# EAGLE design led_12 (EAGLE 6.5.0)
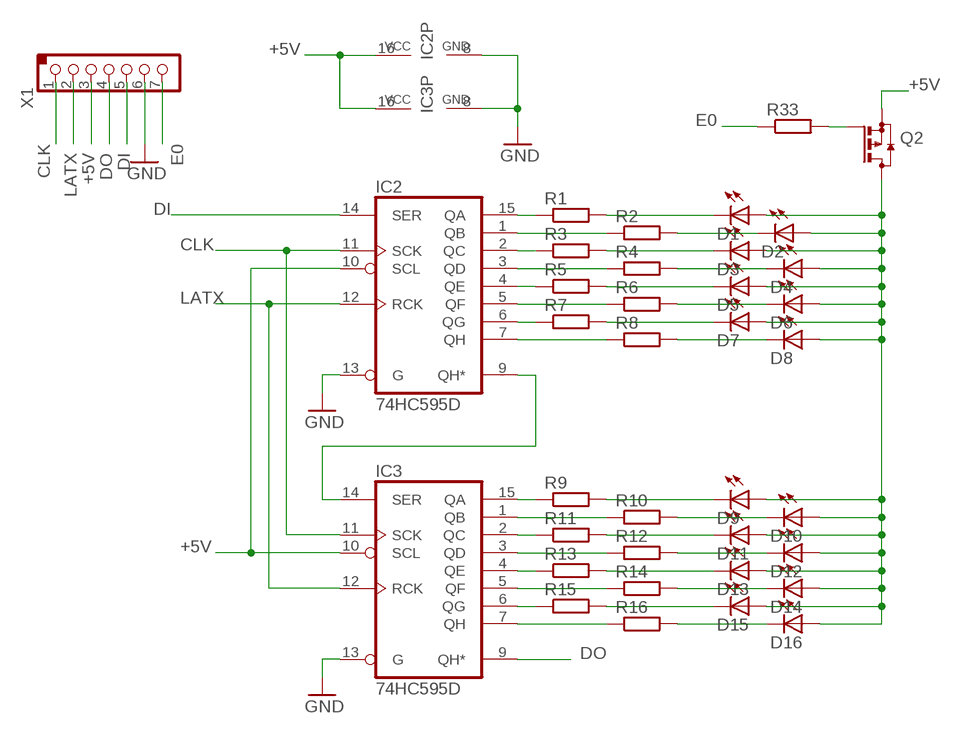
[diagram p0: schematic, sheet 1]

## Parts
D1  LED-SH  [LED5MM_SH]
D2  LED-SH  [LED5MM_SH]
D3  LED-SH  [LED5MM_SH]
D4  LED-SH  [LED5MM_SH]
D5  LED-SH  [LED5MM_SH]
D6  LED-SH  [LED5MM_SH]
D7  LED-SH  [LED5MM_SH]
D8  LED-SH  [LED5MM_SH]
D9  LED-SH  [LED5MM_SH]
D10  LED-SH  [LED5MM_SH]
D11  LED-SH  [LED5MM_SH]
D12  LED-SH  [LED5MM_SH]
D13  LED-SH  [LED5MM_SH]
D14  LED-SH  [LED5MM_SH]
D15  LED-SH  [LED5MM_SH]
D16  LED-SH  [LED5MM_SH]
IC2  74HC595D  [SO16]
IC3  74HC595D  [SO16]
Q2  BSS84  [SOT23]
R1  R_EU-0805  [SMD_0805]
R2  R_EU-0805  [SMD_0805]
R3  R_EU-0805  [SMD_0805]
R4  R_EU-0805  [SMD_0805]
R5  R_EU-0805  [SMD_0805]
R6  R_EU-0805  [SMD_0805]
R7  R_EU-0805  [SMD_0805]
R8  R_EU-0805  [SMD_0805]
R9  R_EU-0805  [SMD_0805]
R10  R_EU-0805  [SMD_0805]
R11  R_EU-0805  [SMD_0805]
R12  R_EU-0805  [SMD_0805]
R13  R_EU-0805  [SMD_0805]
R14  R_EU-0805  [SMD_0805]
R15  R_EU-0805  [SMD_0805]
R16  R_EU-0805  [SMD_0805]
R33  R_EU-1206  [SMD_1206]
X1  PINH_1X7/2  [1X7/2,0]

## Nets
+5V: IC2.10(SCL) IC2.16(VCC) IC3.10(SCL) IC3.16(VCC) Q2.2(S) X1.3
CLK: IC2.11(SCK) IC3.11(SCK) X1.1
DI: IC2.14(SER) X1.5
DO: IC3.9(QH*) X1.4
E0: R33.1 X1.7
GND: IC2.8(GND) IC2.13(G) IC3.8(GND) IC3.13(G) X1.6
LATX: IC2.12(RCK) IC3.12(RCK) X1.2
N$26: IC2.9(QH*) IC3.14(SER)
N$27: IC2.15(QA) R1.1
N$28: IC2.1(QB) R2.1
N$29: IC2.2(QC) R3.1
N$30: IC2.3(QD) R4.1
N$31: IC2.4(QE) R5.1
N$32: IC2.5(QF) R6.1
N$33: IC2.6(QG) R7.1
N$34: IC2.7(QH) R8.1
N$35: D1.C R1.2
N$36: D2.C R2.2
N$37: D3.C R3.2
N$38: D4.C R4.2
N$39: D5.C R5.2
N$40: D6.C R6.2
N$41: D7.C R7.2
N$42: D8.C R8.2
N$43: IC3.15(QA) R9.1
N$44: D9.C R9.2
N$45: IC3.1(QB) R10.1
N$46: D10.C R10.2
N$47: IC3.2(QC) R11.1
N$48: D11.C R11.2
N$49: IC3.3(QD) R12.1
N$50: D12.C R12.2
N$51: IC3.4(QE) R13.1
N$52: D13.C R13.2
N$53: IC3.5(QF) R14.1
N$54: D14.C R14.2
N$55: IC3.6(QG) R15.1
N$56: D15.C R15.2
N$57: IC3.7(QH) R16.1
N$58: D16.C R16.2
N$72: D1.A D2.A D3.A D4.A D5.A D6.A D7.A D8.A D9.A D10.A D11.A D12.A D13.A D14.A D15.A D16.A Q2.3(D)
N$73: Q2.1(G) R33.2

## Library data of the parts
D1-D16 = _dpa222:LED
IC2 IC3 = 74xx-eu:74*595: 8-bit SHIFT REGISTER, output latch
Q2 = transistor-small-signal:BSS84: P-CHANNEL MOS FET
R1-R16 R33 = _dpa222:R_EU
X1 = _dpa222:PINH_1X7/2

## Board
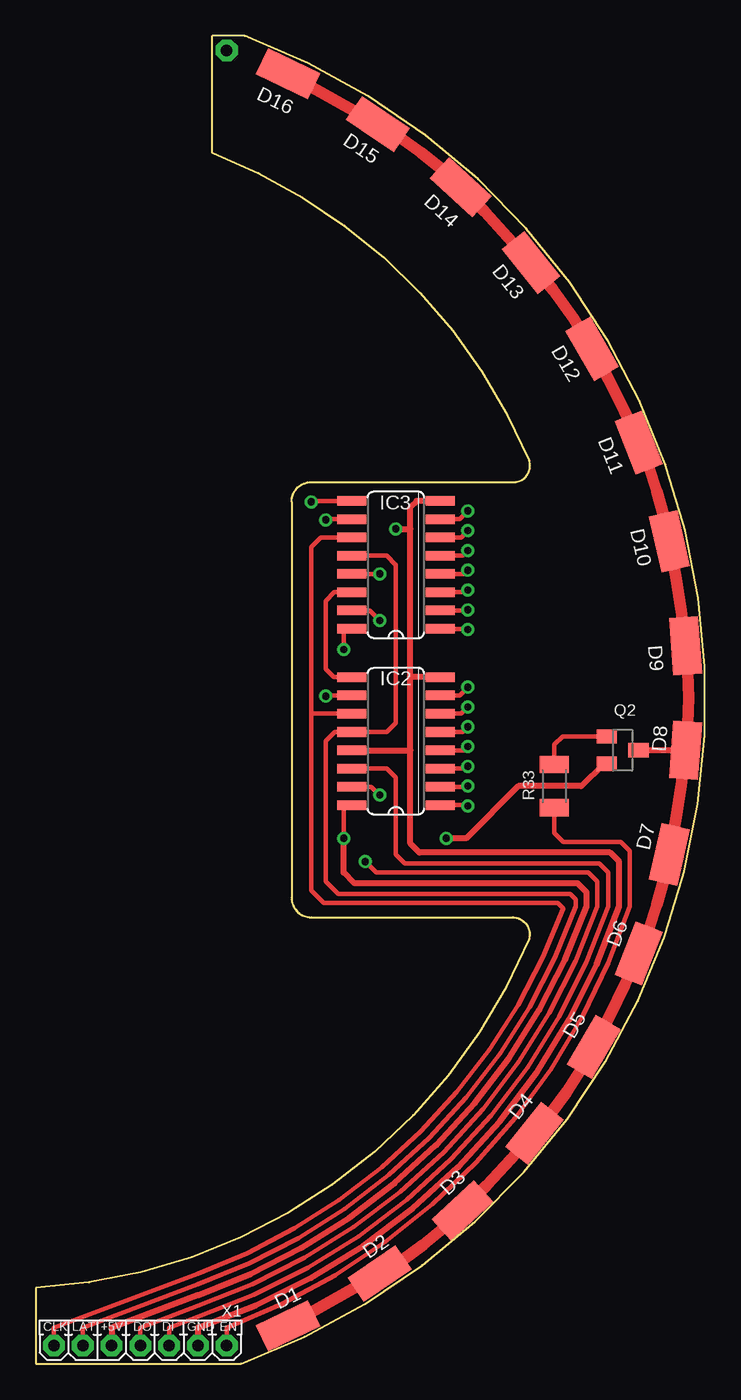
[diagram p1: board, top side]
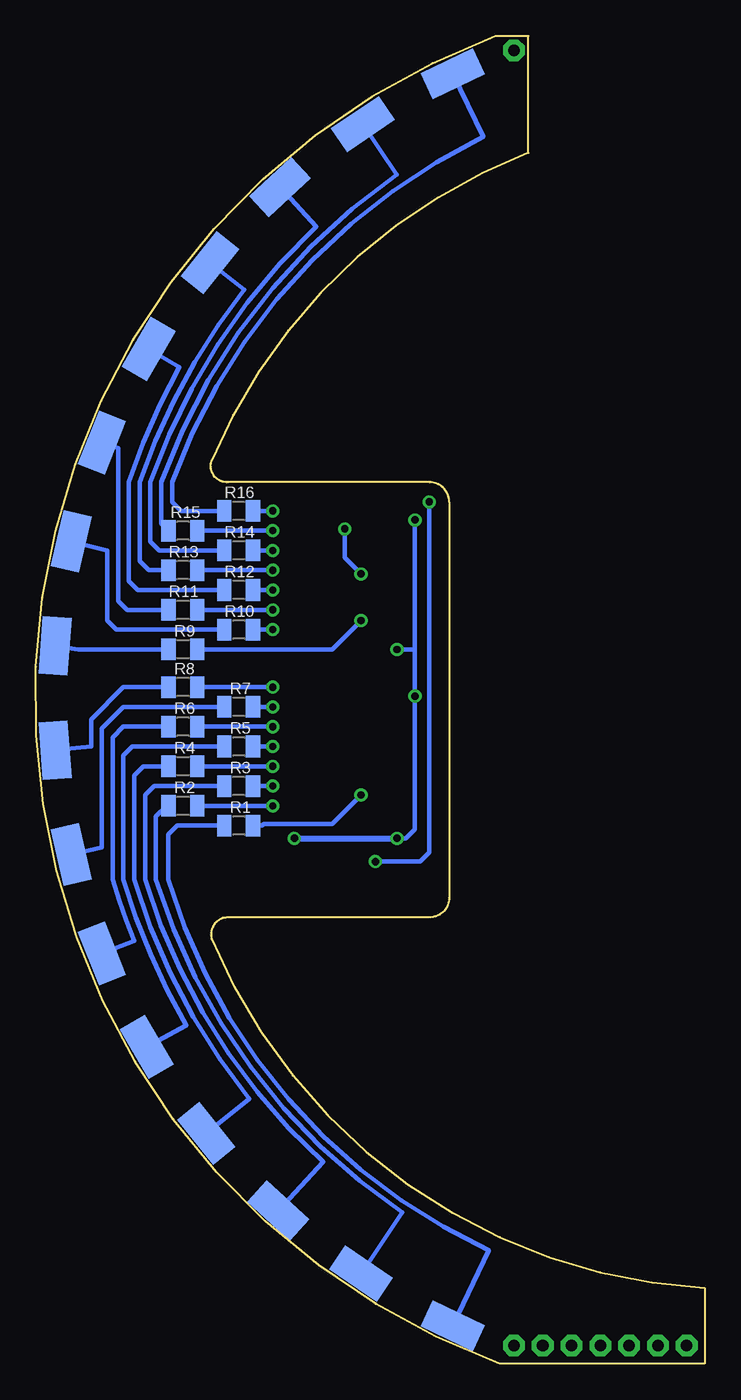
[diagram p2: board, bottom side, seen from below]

Size 46.45 x 92.25 mm. Coordinates in mm from the lower left corner, seen from the top.
Outline: 14.25,0 arc139 14.5,92.25 12.25,92.25 12.25,84.12 arc-46 34.25,62.75 arc-113 33.12,61.25 19.12,61.25 arc90 17.75,59.88 17.75,32.38 arc90 19.12,31 33.12,31 arc-106 34.25,29.5 arc-64 0,5.25 0,0 14.25,0
Copper layers (1*16): Top 0.035mm / dielectric 1.5mm / Bottom 0.035mm
Design rules "default *": minimum track width 10mil, minimum drill 24mil, track to track 8mil, track to pad 8mil, pad to pad 8mil, via to via 8mil, smd to smd 8mil, copper to edge 40mil, drill to drill 8mil, minimum pad ring 10mil, minimum via ring 8mil, stop-mask expansion 4mil, vias tented up to drill 0mil, thermal gap 10mil

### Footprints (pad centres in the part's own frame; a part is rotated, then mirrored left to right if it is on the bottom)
LED5MM_SH = smd 2 x 4: A 0,0 | smd 2 x 4 bottom: C 0,0
SO16 = smd 0.66 x 2.032: 1 -4.445,-3.073; 2 -3.175,-3.073; 3 -1.905,-3.073; 4 -0.635,-3.073; 5 0.635,-3.073; 6 1.905,-3.073; 7 3.175,-3.073; 8 4.445,-3.073; 9 4.445,3.073; 10 3.175,3.073; 11 1.905,3.073; 12 0.635,3.073; 13 -0.635,3.073; 14 -1.905,3.073; 15 -3.175,3.073; 16 -4.445,3.073
SOT23 = smd 1 x 1.4: 1 -0.95,-1.1; 2 0.95,-1.1; 3 0,1.1
SMD_0805 = smd 1 x 1.5: 1 -1,0; 2 1,0
SMD_1206 = smd 1.2 x 2: 1 -1.5,0; 2 1.5,0
1X7/2,0 = drill 0.8 pad 1.5 octagon: 1 -6,0; 2 -4,0; 3 -2,0; 4 0,0; 5 2,0; 6 4,0; 7 6,0

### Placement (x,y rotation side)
D1  17.5,2.62 295.5 top
D2  23.88,6.25 304.1 top
D3  29.62,10.62 312.7 top
D4  34.62,16 321.3 top
D5  38.75,22 329.9 top
D6  41.88,28.5 338.5 top
D7  44,35.38 347.1 top
D8  45.12,42.62 355.7 top
D9  45.12,49.88 4.3 top
D10  44,57.12 12.9 top
D11  41.88,64 21.5 top
D12  38.62,70.5 30.1 top
D13  34.38,76.5 38.7 top
D14  29.5,81.75 47.3 top
D15  23.75,86.12 55.9 top
D16  17.5,89.62 64.5 top
IC2  25,43.25 90 top
IC3  25,55.5 90 top
Q2  40.75,42.62 270 top
R1  32.38,37.38 180 bottom
R2  36.25,38.75 180 bottom
R3  32.38,40.12 180 bottom
R4  36.25,41.5 180 bottom
R5  32.38,42.88 180 bottom
R6  36.25,44.25 180 bottom
R7  32.38,45.62 180 bottom
R8  36.25,47 180 bottom
R9  36.25,49.62 180 bottom
R10  32.38,51 180 bottom
R11  36.25,52.38 180 bottom
R12  32.38,53.75 180 bottom
R13  36.25,55.12 180 bottom
R14  32.38,56.5 180 bottom
R15  36.25,57.88 180 bottom
R16  32.38,59.25 180 bottom
R33  36,40.12 90 top
X1  7.25,1.25 0 top

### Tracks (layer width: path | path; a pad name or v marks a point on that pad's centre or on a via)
+5V  (via drill 0.5)
  Top 0.305: v21.38,36.5 21.38,38.8 IC2.16 | IC3.10 20.12,58.67 v20.12,58.62 | IC2.10 20.12,46.42 v20.12,46.38 | IC3.16 21.38,51.05 v21.38,49.62 | 39.8,41.67 Q2.2 39.42,41.67
  Top 0.406: X1.3 5.25,2.5 11.25,4.75 arc51 38.25,31.75 38.25,32.75 37.62,33.38 22.12,33.38 21.38,34.12 v21.38,36.5 | 39.42,41.67 37.88,40.12 33.5,40.12 29.88,36.5 v28.5,36.5
  Bottom 0.305: v20.12,58.62 20.12,49.62 | 20.12,49.62 v20.12,46.38 20.12,37.12 20.75,36.5 v21.38,36.5 | v21.38,49.62 20.12,49.62
  Bottom 0.406: v28.5,36.5 v21.38,36.5
CLK
  Top 0.305: 11.25,6.25 arc50 36.62,31.62 | 11.25,6.25 1.25,2.5 X1.1 | 36.62,31.62 36.25,32 20,32 19.12,32.88 19.12,45.16 | IC2.11 19.12,45.16 | 19.12,45.16 19.12,56.75 19.78,57.41 IC3.11 | 11.25,6.25 arc50 36.62,31.62
  Bottom 0.305: X1.1 1.25,1.75
DI
  Top 0.305: X1.5 9.25,2.5 11.25,3.25 arc53 39.75,31.75 39.75,34.12 39.12,34.75 25.62,34.75 25,35.38 25,40.72 24.38,41.34 IC2.14
DO  (via drill 0.5)
  Top 0.305: X1.4 7.25,2.5 11.25,4 arc52 39,31.75 39,33.5 38.38,34.12 23.62,34.12 v22.88,34.88 | IC3.9 19.12,59.95 v19.12,59.88
  Bottom 0.305: v22.88,34.88 19.75,34.88 19.12,35.5 v19.12,59.88
E0
  Top 0.305: X1.7 13.25,2.5 arc51 41.25,31.75 41.25,35.62 40.62,36.25 36.62,36.25 36,36.88 R33.1
GND  (via drill 0.5)
  Top 0.305: IC3.13 v23.88,54.87 v23.88,54.88 | 28.13,60 IC3.8
  Top 0.406: X1.6 11.25,2.5 arc53 40.5,31.75 40.5,34.88 39.88,35.5 26.62,35.5 26,36.12 26,42.62 | 26,42.62 26,47.7 | 26,47.7 26,58 | 26,58 26,59.5 26.45,59.95 IC3.8 | IC2.8 26,47.7 | IC2.13 26,42.62 | v25,58 26,58
  Bottom 0.305: v23.88,54.88 25,56 v25,58
LATX
  Top 0.305: X1.2 3.25,2.5 11.25,5.5 arc51 37.5,31.75 37.5,32.25 37.12,32.62 21,32.62 20.12,33.5 20.12,43.26 | 20.14,43.26 20.12,43.26 | IC2.12 | IC3.12 24.36,56.13 25,55.5 | 25,55.5 25,55.51 | 25,55.5 25,44.51 24.38,43.88 IC2.12 | IC2.12 20.75,43.88 20.12,43.26
N$26
  Top 0.305: IC3.14 20.72,53.59 20.12,53 20.12,48.25 20.68,47.7 IC2.9
N$27  (via drill 0.5)
  Top 0.305: IC2.15 23.3,40.08 v23.88,39.5
  Bottom 0.305: v23.88,39.5 25.88,37.5 30.62,37.5 30.75,37.38 R1.1
N$28  (via drill 0.5)
  Top 0.305: IC2.1 30,38.8 v30,38.75
  Bottom 0.305: v30,38.75 R2.1
N$29  (via drill 0.5)
  Top 0.305: IC2.2 30,40.08 v30,40.12
  Bottom 0.305: v30,40.12 R3.1
N$30  (via drill 0.5)
  Top 0.305: IC2.3 29.84,41.34 v30,41.5
  Bottom 0.305: v30,41.5 R4.1
N$31  (via drill 0.5)
  Top 0.305: IC2.4 29.74,42.62 v30,42.88
  Bottom 0.305: v30,42.88 R5.1
N$32  (via drill 0.5)
  Top 0.305: IC2.5 29.63,43.88 v30,44.25
  Bottom 0.305: v30,44.25 R6.1
N$33  (via drill 0.5)
  Top 0.305: IC2.6 29.53,45.16 v30,45.62
  Bottom 0.305: v30,45.62 R7.1
N$34  (via drill 0.5)
  Top 0.305: IC2.7 29.42,46.42 v30,47
  Bottom 0.305: v30,47 R8.1
N$35
  Bottom 0.305: D1.C 15,7.88 arc49 37.25,33.62 37.25,36.75 36.62,37.38 R1.2
N$36
  Bottom 0.305: D2.C 21,10.5 arc39 38.12,33.62 38.12,38 37.38,38.75 R2.2 37.12,38.62
N$37
  Bottom 0.305: D3.C 26.5,14 arc31 38.88,33.62 38.88,39.5 38.25,40.12 R3.2
N$38
  Bottom 0.305: D4.C 31.62,18.38 arc22 39.62,33.62 39.62,40.88 39,41.5 R4.2
N$39
  Bottom 0.305: D5.C 36,23.5 arc14 40.38,33.62 40.38,42.25 39.75,42.88 R5.2
N$40
  Bottom 0.305: D6.C 39.62,29.38 arc6 41.12,33.62 41.12,43.5 40.38,44.25 R6.2
N$41
  Bottom 0.305: D7.C 41.88,35.88 41.88,44.12 40.38,45.62 R7.2
N$42
  Bottom 0.305: R8.2 40.38,47 42.62,44.75 42.62,42.88 D8.C
N$43  (via drill 0.5)
  Top 0.305: IC3.15 23.18,52.33 v23.88,51.62
  Bottom 0.305: v23.88,51.62 25.88,49.62 R9.1
N$44
  Bottom 0.305: R9.2 43.5,49.62 D9.C
N$45  (via drill 0.5)
  Top 0.305: IC3.1 29.95,51.05 v30,51
  Bottom 0.305: v30,51 R10.1
N$46
  Bottom 0.305: R10.2 40.88,51 41.5,51.62 41.5,56.5 D10.C
N$47  (via drill 0.5)
  Top 0.305: IC3.2 29.95,52.33 v30,52.38
  Bottom 0.305: v30,52.38 R11.1
N$48
  Bottom 0.305: R11.2 40.12,52.38 40.75,53 40.75,63.62 D11.C
N$49  (via drill 0.5)
  Top 0.305: IC3.3 29.84,53.59 v30,53.75
  Bottom 0.305: v30,53.75 R12.1
N$50
  Bottom 0.305: R12.2 39.38,53.75 40,54.38 40,61.25 arc11 36.5,69.25 D12.C
N$51  (via drill 0.5)
  Top 0.305: IC3.4 29.74,54.87 v30,55.12
  Bottom 0.305: v30,55.12 R13.1
N$52
  Bottom 0.305: R13.2 38.62,55.12 39.25,55.75 39.25,61.25 arc19 32,74.62 D13.C
N$53  (via drill 0.5)
  Top 0.305: IC3.5 29.63,56.13 v30,56.5
  Bottom 0.305: v30,56.5 R14.1
N$54
  Bottom 0.305: R14.2 37.88,56.5 38.5,57.12 38.5,61.25 arc27 27,79 D14.C
N$55  (via drill 0.5)
  Top 0.305: IC3.6 29.53,57.41 v30,57.88
  Bottom 0.305: v30,57.88 R15.1
N$56
  Bottom 0.305: D15.C 21.38,82.62 arc-36 37.75,61.25 37.75,58.38 R15.2
N$57  (via drill 0.5)
  Top 0.305: IC3.7 29.42,58.67 v30,59.25
  Bottom 0.305: v30,59.25 R16.1
N$58
  Bottom 0.305: R16.2 36.38,59.25 37,59.88 37,61.25 arc44 15.38,85.25 D16.C
N$70  (via drill 0.8 pad 1.5)
  other vias: 13.25,91.25
N$72
  Top 0.406: Q2.3 D8.A
  Top 0.813: D16.A D15.A arc-16 D14.A arc-4 D13.A arc-11 D12.A arc-6 D11.A arc-13 D10.A arc-4 D9.A arc-14 D8.A arc-4 D7.A arc-13 D6.A arc-4 D5.A arc-13 D4.A arc-3 D3.A arc-16 D2.A arc1 D1.A
N$73
  Top 0.305: Q2.1 36.58,43.58 36,43 R33.2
